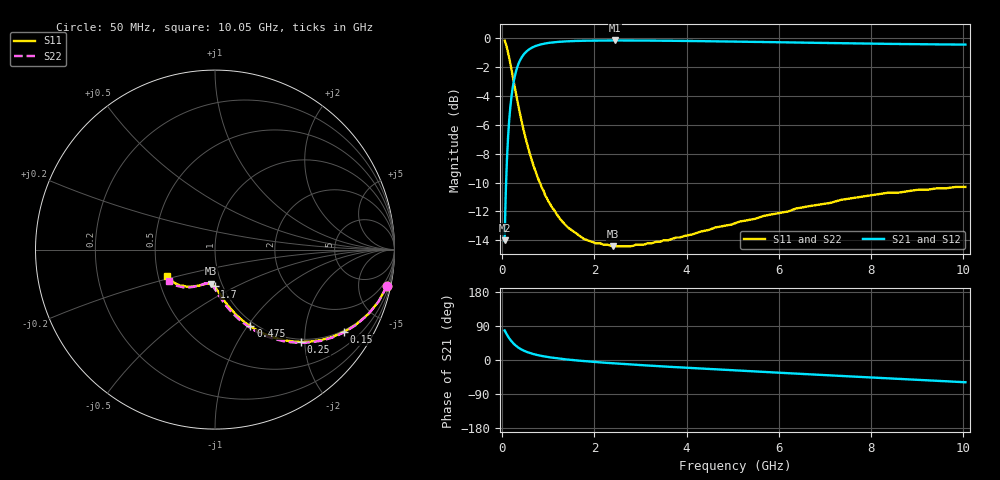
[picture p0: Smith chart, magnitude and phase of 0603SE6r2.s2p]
! AVX Thin Film Operation		Date: August 2001
! Description: Accu-P® Series, Thin Film, SMD, RF Capacitor
! Part Number: 06035J6R2BBT
! 50 MHz  -  10.05 GHz
! Serial Measurements
# mhz S db R 50
!	S11		S21		S12		S22
!	dB	Phase	dB	Phase	dB	Phase	dB	Phase
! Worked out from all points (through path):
!   401 points, 50 MHz to 10.05 GHz, reference 50 ohm
!   highest |S21| = -0.17 dB at 2.45 GHz (marker M1); lowest = -14.0 dB at 50 MHz (marker M2)
!   group delay of S21, straight-line fit = 22.5 ps
!   lowest |S11| = -14.4 dB at 2.4 GHz (marker M3), VSWR 1.47, Z = 44.4 - j17.4 ohm
!   |S11| at or under -10 dB: 815.1 MHz to end of sweep
!   |S22| runs from -14.4 to -0.2 dB; largest |S21 - S12| = 0
!   S11 on the Smith chart (normalised r, x): 50 MHz: 0.94, -9.50; 150 MHz: 0.94, -3.18; 250 MHz: 0.94, -1.92; 475 MHz: 0.94, -1.03; 1.7 GHz: 0.91, -0.39; 10.05 GHz: 0.56, -0.18
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50  -0.18 -11.9  -14.00 78.1  -14.00 78.1  -0.18 -12.0
100  -0.67 -22.9  -8.47 67.0  -8.47 67.0  -0.67 -23.1
125  -1.01 -27.9  -6.86 62.0  -6.86 62.0  -1.01 -28.2
150  -1.38 -32.4  -5.66 57.3  -5.66 57.3  -1.38 -32.8
200  -2.19 -40.4  -4.02 49.4  -4.02 49.4  -2.19 -40.9
250  -3.05 -47.0  -2.98 42.7  -2.98 42.7  -3.05 -47.6
300  -3.90 -52.4  -2.27 37.2  -2.27 37.2  -3.90 -53.1
350  -4.72 -56.9  -1.79 32.6  -1.79 32.6  -4.72 -57.7
475  -6.54 -65.2  -1.09 24.2  -1.09 24.2  -6.54 -66.3
575  -7.76 -69.9  -0.80 19.4  -0.80 19.4  -7.76 -71.2
675  -8.81 -73.4  -0.62 15.7  -0.62 15.7  -8.81 -75.0
975  -11.13 -80.8  -0.35 8.1  -0.35 8.1  -11.13 -82.8
1325  -12.78 -86.3  -0.24 2.4  -0.24 2.4  -12.78 -88.6
1700  -13.74 -90.7  -0.19 -2.1  -0.19 -2.1  -13.72 -93.1
1725  -13.80 -91.0  -0.19 -2.4  -0.19 -2.4  -13.75 -93.3
2400  -14.40 -97.3  -0.17 -8.6  -0.17 -8.6  -14.40 -99.5
2450  -14.40 -97.7  -0.17 -9.1  -0.17 -9.1  -14.40 -99.9
3400  -14.10 -105.0  -0.18 -16.3  -0.18 -16.3  -14.10 -106.8
5050  -12.82 -117.4  -0.25 -27.5  -0.25 -27.5  -12.76 -117.4
6725  -11.60 -129.0  -0.33 -38.1  -0.33 -38.1  -11.60 -127.0
8400  -10.70 -140.1  -0.41 -48.6  -0.41 -48.6  -10.69 -136.2
10050  -10.30 -150.8  -0.45 -58.7  -0.45 -58.7  -10.22 -145.8
